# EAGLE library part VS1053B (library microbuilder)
VS1053b Audio Codec - Ogg Vorbis/MP3/AAC/WMA/FLAC/MIDI
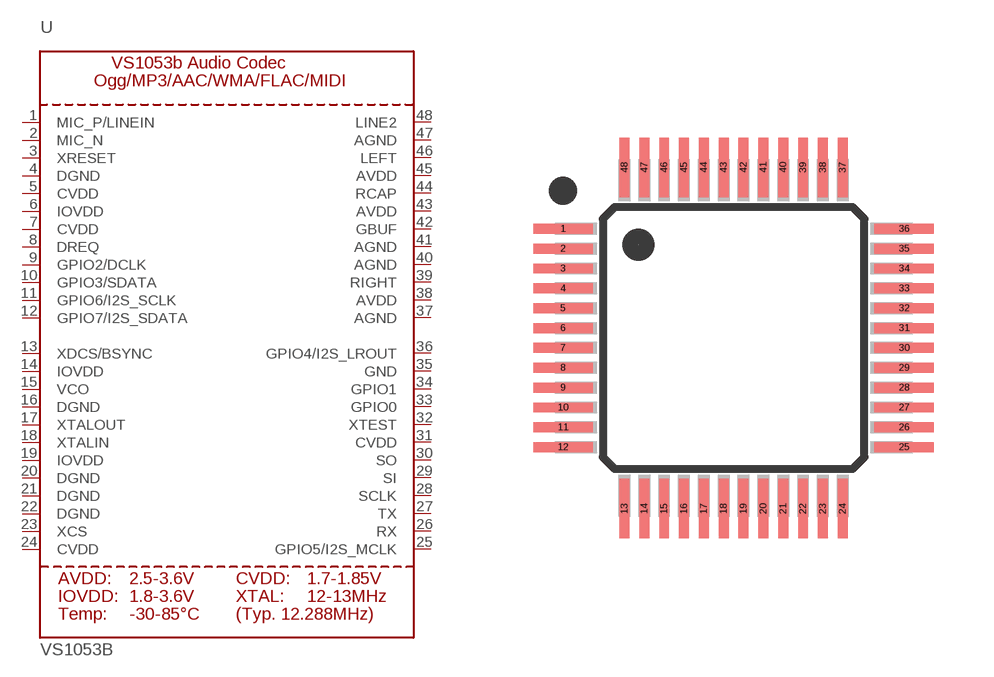
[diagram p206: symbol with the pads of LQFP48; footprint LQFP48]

Designator prefix U

## VS1053B  [LQFP48]
1  MIC_P/LINEIN
2  MIC_N
3  XRESET
4  DGND  sup
5  CVDD  sup
6  IOVDD  sup
7  CVDD  sup
8  DREQ
9  GPIO2/DCLK
10  GPIO3/SDATA
11  GPIO6/I2S_SCLK
12  GPIO7/I2S_SDATA
13  XDCS/BSYNC
14  IOVDD  sup
15  VCO
16  DGND  sup
17  XTALOUT  out
18  XTALIN  in
19  IOVDD  sup
20  DGND  sup
21  DGND  sup
22  DGND  sup
23  XCS
24  CVDD  sup
25  GPIO5/I2S_MCLK
26  RX
27  TX
28  SCLK
29  SI
30  SO
31  CVDD  sup
32  XTEST
33  GPIO0
34  GPIO1
35  GND  sup
36  GPIO4/I2S_LROUT
37  AGND  sup
38  AVDD  sup
39  RIGHT
40  AGND  sup
41  AGND  sup
42  GBUF
43  AVDD  sup
44  RCAP
45  AVDD  sup
46  LEFT
47  AGND  sup
48  LINE2

## Footprint LQFP48 (pad centres in mm)
smd 1.5 x 0.25: 1 -4.3,2.75; 2 -4.3,2.25; 3 -4.3,1.75; 4 -4.3,1.25; 5 -4.3,0.75; 6 -4.3,0.25; 7 -4.3,-0.25; 8 -4.3,-0.75; 9 -4.3,-1.25; 10 -4.3,-1.75; 11 -4.3,-2.25; 12 -4.3,-2.75; 25 4.3,-2.75; 26 4.3,-2.25; 27 4.3,-1.75; 28 4.3,-1.25; 29 4.3,-0.75; 30 4.3,-0.25; 31 4.3,0.25; 32 4.3,0.75; 33 4.3,1.25; 34 4.3,1.75; 35 4.3,2.25; 36 4.3,2.75
smd 0.25 x 1.5: 13 -2.75,-4.3; 14 -2.25,-4.3; 15 -1.75,-4.3; 16 -1.25,-4.3; 17 -0.75,-4.3; 18 -0.25,-4.3; 19 0.25,-4.3; 20 0.75,-4.3; 21 1.25,-4.3; 22 1.75,-4.3; 23 2.25,-4.3; 24 2.75,-4.3; 37 2.75,4.3; 38 2.25,4.3; 39 1.75,4.3; 40 1.25,4.3; 41 0.75,4.3; 42 0.25,4.3; 43 -0.25,4.3; 44 -0.75,4.3; 45 -1.25,4.3; 46 -1.75,4.3; 47 -2.25,4.3; 48 -2.75,4.3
